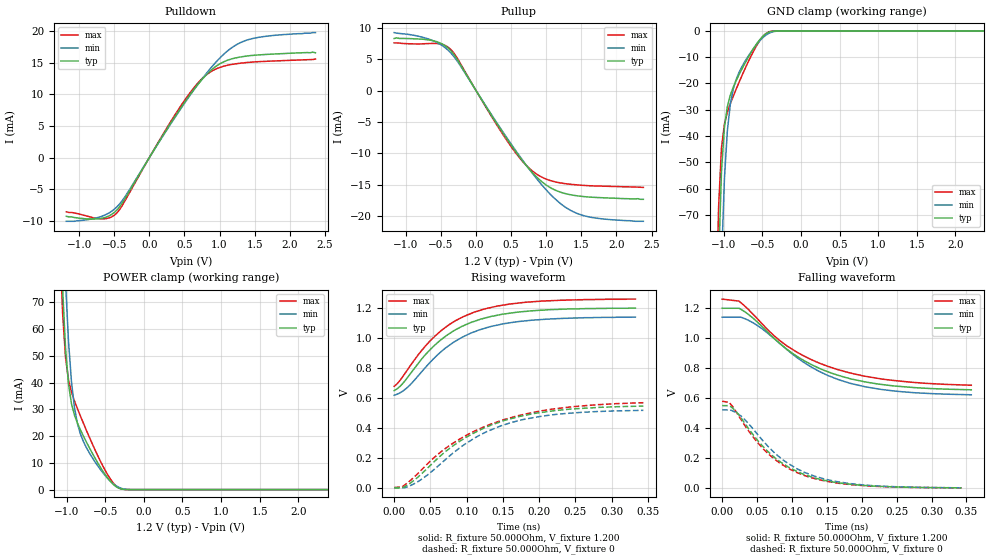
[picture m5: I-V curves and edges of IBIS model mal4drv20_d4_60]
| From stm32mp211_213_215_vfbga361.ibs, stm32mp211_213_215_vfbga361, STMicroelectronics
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[Model] mal4drv20_d4_60
Model_type   I/O
Polarity   Non-Inverting
Enable   Active-High
C_comp   1.838pF   1.835pF   1.848pF
C_comp_pullup   938.881fF   931.604fF   947.115fF
C_comp_pulldown 782.410fF   779.859fF   796.520fF
Vinh = 668.000mV
Vinl = 532.000mV
Vmeas = 600.000mV
Vref = 600.000mV
Rref = 50Ohms
Cref = 0pF
[Model Spec]
Vinh   668.000mV   638.000mV   698.000mV
Vinl   532.000mV   502.000mV   562.000mV
Vmeas   600.000mV   570.000mV   630.000mV
Vref   600.000mV   570.000mV   630.000mV
D_overshoot_ampl_h 0.24 NA   NA
D_overshoot_ampl_l 0.24 NA   NA
D_overshoot_area_l 300.000m NA   NA
D_overshoot_area_h 300.000m NA   NA
[Receiver Thresholds]
Vth = 600.000mV
Vth_min = 570.000mV
Vth_max = 630.000mV
Vinh_ac = 68.000mV
Vinh_dc = 68.000mV
Vinl_ac = -68.000mV
Vinl_dc = -68.000mV
Tslew_ac = 5.000ns
Threshold_sensitivity = 0.5
Reference_supply Pullup_ref
[Temperature Range]   25.000   125.000   -40.000
[Voltage Range]   1.200V   1.140V   1.260V
[GND Clamp Reference]   0.00V   0.00V   0.00V
[C Comp Corner]
| variable   typ   min   max
C_comp 1.848pF   1.838pF   1.835pF
C_comp_pullup 938.881fF   947.115fF   931.604fF
C_comp_pulldown 779.859fF   796.520fF   782.410fF
[Pulldown Reference]   0.00V   0.00V   0.00V
[POWER Clamp Reference]   1.200V   1.140V   1.260V
[Pullup Reference]   1.200V   1.140V   1.260V
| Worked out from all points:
|   slope of the pulldown table from 0 to 0.18 V, typ, clamps not added: 55 ohm
|   slope of the pullup table from 0 to 0.18 V, typ, clamps not added: 55.5 ohm
|   GND clamp passes 1 mA (typ) near -0.45 V on its own axis
|   POWER clamp passes 1 mA (typ) near -0.35 V on its own axis
|   rising waveform, R_fixture 50.000Ohm, V_fixture 1.200: 20-80 % time 77ps typ, 78.7ps min, 76.6ps max; typ from 0.648 V to 1.2 V
|   rising waveform, R_fixture 50.000Ohm, V_fixture 0: 20-80 % time 103ps typ, 96.8ps min, 114ps max; typ from -0.002 V to 0.544 V
|   falling waveform, R_fixture 50.000Ohm, V_fixture 1.200: 20-80 % time 104ps typ, 101ps min, 111ps max; typ from 1.2 V to 0.656 V
|   falling waveform, R_fixture 50.000Ohm, V_fixture 0: 20-80 % time 75.7ps typ, 77.2ps min, 74.7ps max; typ from 0.55 V to 0.001 V
[GND Clamp]
-1.184V   -365mA     -429.3mA   -336.5mA
-1.107V   -152.4mA   -215.7mA   -121.1mA
-1.069V   -88.87mA   -140.5mA   -67.62mA
-1.031V   -53.54mA   -88.39mA   -44.48mA
-992.7mV  -36.7mA    -56.18mA   -35.42mA
-954.6mV  -28.78mA   -37.93mA   -30.92mA
-916.4mV  -24.43mA   -27.89mA   -27.7mA
-840mV    -18.89mA   -18.42mA   -22.12mA
-763.6mV  -14.38mA   -13.51mA   -16.88mA
-572.7mV  -4.818mA   -5.067mA   -5.477mA
-458.2mV  -1.146mA   -1.695mA   -1.103mA
2.367V    25.44nA    625nA      8.401nA
[Power Clamp]
-1.167V   197.6mA    234.2mA    183.1mA
-1.091V   108mA      144mA      94.42mA
-1.053V   75.21mA    107.2mA    65.93mA
-1.015V   52.65mA    77.42mA    49.33mA
-976.4mV  39.37mA    55.31mA    41.02mA
-938.2mV  32.15mA    40.29mA    36.48mA
-900mV    27.91mA    30.75mA    33.22mA
-823.6mV  22.42mA    20.91mA    27.62mA
-632.7mV  11.76mA    10.36mA    14.83mA
-365.4mV  1.178mA    1.496mA    1.508mA
-212.7mV  14.35uA    76.22uA    9.056uA
2.384V    -16.74nA   -562.7nA   -5.86nA
[Pulldown]
-1.184V   -9.3mA     -10.1mA    -8.6mA
-725.5mV  -9.7mA     -9.48mA    -9.67mA
-572.7mV  -9.232mA   -8.763mA   -9.563mA
-458.2mV  -8.26mA    -7.767mA   -8.717mA
-343.6mV  -6.433mA   -6.146mA   -6.776mA
152.7mV   2.782mA    2.701mA    2.914mA
496.4mV   8.659mA    8.523mA    8.969mA
725.5mV   12.04mA    12.08mA    12.22mA
954.5mV   14.5mA     15.19mA    14.06mA
1.184V    15.66mA    17.48mA    14.77mA
1.413V    16.12mA    18.69mA    15.08mA
2.367V    16.6mA     19.8mA     15.6mA
[Pullup]
-1.167V   8.3mA      9.243mA    7.6mA
-632.7mV  7.99mA     8.035mA    7.514mA
-480mV    7.413mA    7.148mA    7.355mA
-365.4mV  6.417mA    6.064mA    6.608mA
-289.1mV  5.303mA    5.03mA     5.535mA
474.6mV   -8.269mA   -8.093mA   -8.513mA
703.6mV   -11.76mA   -11.7mA    -11.77mA
894.5mV   -14.09mA   -14.45mA   -13.51mA
1.2V      -16.15mA   -17.95mA   -14.68mA
1.467V    -16.78mA   -19.66mA   -15.03mA
1.773V    -17.03mA   -20.38mA   -15.2mA
2.384V    -17.3mA    -20.8mA    -15.4mA
[Ramp]
R_load=50.000Ohm
dV/dt_r   329.910mV/92.000ps  312.898mV/89.500ps  347.520mV/99.000ps
dV/dt_f   329.910mV/92.500ps  312.898mV/91.000ps  347.520mV/96.500ps
[Rising waveform]
R_fixture=50.000Ohm
V_fixture=1.200
V_fixture_min=1.140
V_fixture_max=1.260
0s        648.2mV    617mV      676.7mV
9ps       680.8mV    635.7mV    722mV
19ps      739.5mV    672.4mV    791.7mV
40ps      871mV      785.1mV    928.2mV
56ps      951.6mV    869mV      1.011V
81ps      1.044V     968mV      1.104V
111ps     1.111V     1.041V     1.173V
149ps     1.158V     1.093V     1.218V
191ps     1.181V     1.119V     1.241V
333ps     1.199V     1.139V     1.259V
[Rising waveform]
R_fixture=50.000Ohm
V_fixture=0
0s        -1.966mV   -524.6uV   -343uV
11ps      -1.966mV   -524.6uV   5.667mV
31ps      62.44mV    34.64mV    85.63mV
57ps      181.6mV    128.7mV    208.7mV
87ps      298.5mV    252.9mV    314.3mV
116ps     379.2mV    345mV      389.2mV
151ps     447.1mV    418.2mV    453.2mV
177ps     479.4mV    453.6mV    487.1mV
219ps     512.8mV    486.8mV    524.5mV
344ps     544.4mV    516mV      566.9mV
[Falling waveform]
R_fixture=50.000Ohm
V_fixture=1.200
V_fixture_min=1.140
V_fixture_max=1.260
0s        1.201V     1.141V     1.262V
24ps      1.201V     1.141V     1.249V
44ps      1.136V     1.105V     1.163V
71ps      1.016V     1.012V     1.032V
93ps      926.1mV    924mV      949.1mV
120ps     844mV      830.2mV    875.3mV
148ps     782.9mV    759.2mV    818.6mV
184ps     729.4mV    698.9mV    767.9mV
233ps     689.2mV    655.3mV    725.5mV
357ps     656.2mV    622.9mV    686.5mV
[Falling waveform]
R_fixture=50.000Ohm
V_fixture=0
0s        550.4mV    521.7mV    579.9mV
10ps      550.4mV    521.7mV    571.7mV
26ps      475.6mV    484.8mV    465mV
44ps      358mV      396.6mV    342.9mV
66ps      242.3mV    277mV      228.9mV
91ps      151.3mV    174.7mV    141.8mV
114ps     97.21mV    113mV      89.86mV
145ps     52.54mV    61.73mV    48.9mV
198ps     18.77mV    22.03mV    17.25mV
343ps     1.071mV    1.427mV    958.5uV
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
